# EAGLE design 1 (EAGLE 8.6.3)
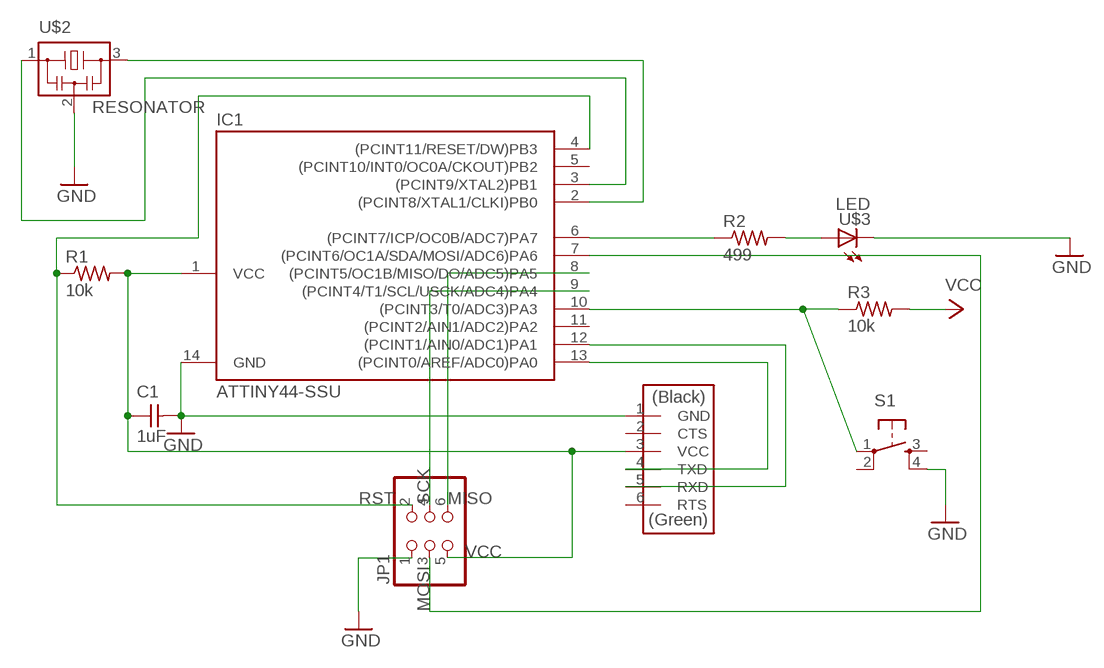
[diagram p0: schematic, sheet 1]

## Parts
C1  1uF  CAP-UNPOLARIZEDFAB  [C1206FAB]
IC1  ATTINY44-SSU  [SOIC14]
JP1  PINHD-2X3-SMD  [2X03SMD]
R1  10k  RES-US1206FAB  [R1206FAB]
R2  499  RES-US1206FAB  [R1206FAB]
R3  10k  RES-US1206FAB  [R1206FAB]
S1  6MM_SWITCH6MM_SWITCH  [6MM_SWITCH]
U$1  FTDI-SMD-HEADER  [1X06SMD]
U$2  RESONATOR  [EFOBM]
U$3  LED  [LED1206]

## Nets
GND: C1.2 IC1.14(GND) JP1.1 S1.4(S1) U$1.1(GND) U$2.2 U$3.2(C)
MISO: IC1.8((PCINT5/OC1B/MISO/DO/ADC5)PA5) JP1.6
MOSI: IC1.7((PCINT6/OC1A/SDA/MOSI/ADC6)PA6) JP1.3
N$1: IC1.2((PCINT8/XTAL1/CLKI)PB0) U$2.3
N$2: IC1.3((PCINT9/XTAL2)PB1) U$2.1
N$4: IC1.13((PCINT0/AREF/ADC0)PA0) U$1.4(TXD)
N$5: IC1.12((PCINT1/AIN0/ADC1)PA1) U$1.5(RXD)
N$6: IC1.6((PCINT7/ICP/OC0B/ADC7)PA7) R2.1
N$7: R2.2 U$3.1(A)
N$8: IC1.10((PCINT3/T0/ADC3)PA3) R3.1 S1.1(P)
RST: IC1.4((PCINT11/RESET/DW)PB3) JP1.2 R1.1
SCK: IC1.9((PCINT4/T1/SCL/USCK/ADC4)PA4) JP1.4
VCC: C1.1 IC1.1(VCC) JP1.5 R1.2 R3.2 U$1.3(VCC)
Unconnected: IC1.5((PCINT10/INT0/OC0A/CKOUT)PB2) IC1.11((PCINT2/AIN1/ADC2)PA2) S1.2(P1) S1.3(S) U$1.2(CTS) U$1.6(RTS)

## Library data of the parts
C1 = fab:CAP-UNPOLARIZED
IC1 = fab:ATTINY44
JP1 = fab:PINHD-2X3-SMD: PIN HEADER
R1-R3 = fab:RES-US: Resistor (US Symbol)
S1 = fab:6MM_SWITCH: OMRON SWITCH
U$1 = fab:FTDI-SMD-HEADER
U$2 = fab:RESONATOR
U$3 = fab:LED: LED

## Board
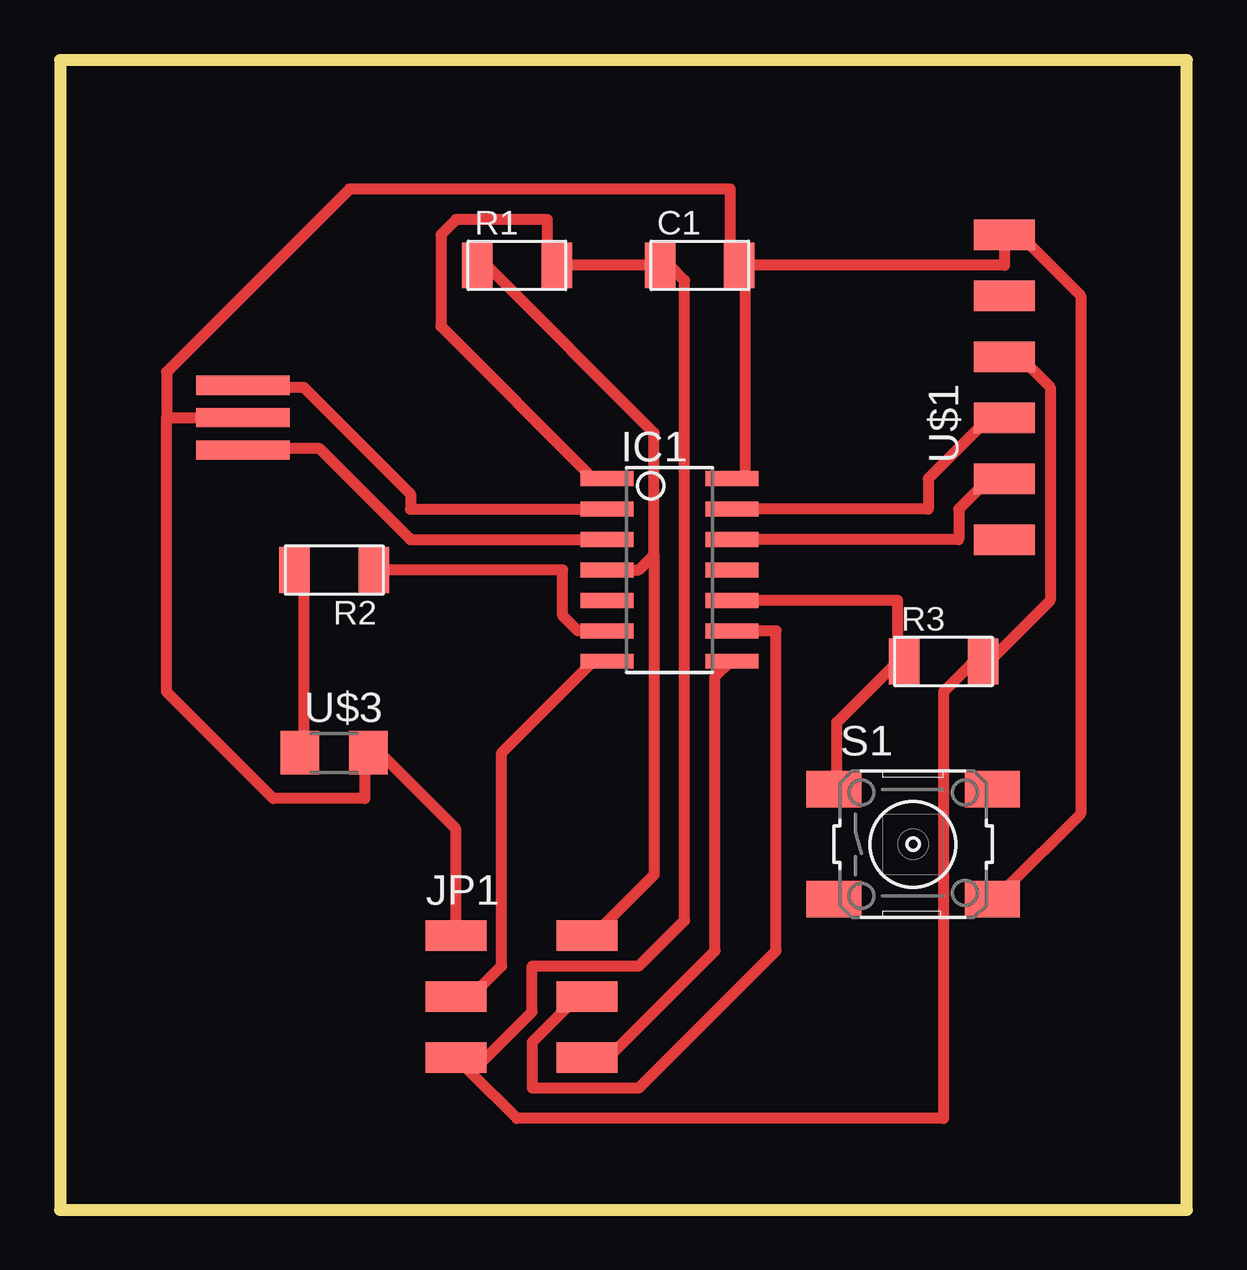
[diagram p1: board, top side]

Size 46.97 x 47.93 mm. Coordinates in mm from the lower left corner, seen from the top.
Outline: 0,0 46.97,0 46.97,47.93 0,47.93 0,0
Copper layers (1*16): Top 0.035mm / dielectric 1.5mm / Bottom 0.035mm
Design rules "default *": minimum track width 16mil, minimum drill 0.35mm, track to track 16mil, track to pad 16mil, pad to pad 16mil, via to via 16mil, smd to smd 16mil, copper to edge 40mil, drill to drill 6mil, minimum pad ring 10mil, minimum via ring 8mil, stop-mask expansion 4mil, vias tented up to drill 0mil, thermal gap 10mil

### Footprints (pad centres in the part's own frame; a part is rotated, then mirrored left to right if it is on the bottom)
C1206FAB = smd 1.27 x 1.905: 1 -1.651,0; 2 1.651,0
SOIC14 = smd 0.61 x 2.21: 1 -3.81,-2.603; 2 -2.54,-2.603; 3 -1.27,-2.603; 4 0,-2.603; 5 1.27,-2.603; 6 2.54,-2.603; 7 3.81,-2.603; 8 3.81,2.603; 9 2.54,2.603; 10 1.27,2.603; 11 0,2.603; 12 -1.27,2.603; 13 -2.54,2.603; 14 -3.81,2.603
2X03SMD = smd 2.54 x 1.27: 1 -2.54,2.54; 2 2.92,2.54; 3 -2.54,0; 4 2.92,0; 5 -2.54,-2.54; 6 2.92,-2.54
R1206FAB = smd 1.27 x 1.905: 1 -1.651,0; 2 1.651,0
6MM_SWITCH = smd 2.286 x 1.524: 1 -3.302,2.286; 2 3.302,2.286; 3 -3.302,-2.286; 4 3.302,-2.286
1X06SMD = smd 2.54 x 1.27: 1 0,6.35; 2 0,3.81; 3 0,1.27; 4 0,-1.27; 5 0,-3.81; 6 0,-6.35
EFOBM = smd 0.8 x 3.9: 1 -1.35,0; 2 0,0; 3 1.35,0
LED1206 = smd 1.6 x 1.803: 1 -1.422,0; 2 1.422,0

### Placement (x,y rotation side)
C1  26.67,39.37 0 top
IC1  25.4,26.67 270 top
JP1  19.05,8.89 0 top
R1  19.05,39.37 0 top
R2  11.43,26.67 180 top
R3  36.83,22.86 0 top
S1  35.56,15.24 0 top
U$1  39.37,34.29 0 top
U$2  7.62,33.02 90 top
U$3  11.43,19.05 0 top

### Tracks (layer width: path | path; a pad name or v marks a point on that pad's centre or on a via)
GND
  Top 0.457: JP1.1 16.51,15.88 13.33,19.05 U$3.2 12.7,19.05 12.7,17.15 8.89,17.15 4.45,21.59 4.45,33.02 | 4.45,33.02 U$2.2 | 28.57,39.37 28.57,30.48 IC1.14 | S1.4 39.37,13.33 42.55,16.51 42.55,38.1 40,40.64 U$1.1 39.37,39.37 28.57,39.37 | 28.57,39.37 C1.2 27.94,39.37 27.94,42.55 12.06,42.55 4.45,34.92 4.45,33.02
MISO
  Top 0.457: JP1.6 22.86,6.35 27.3,10.79 27.3,22.23 27.94,22.86 IC1.8
MOSI
  Top 0.457: JP1.3 17.14,8.89 18.41,10.16 18.41,19.05 22.23,22.86 IC1.7
N$1
  Top 0.457: IC1.2 14.6,29.21 14.6,29.84 10.16,34.29 7.62,34.29 U$2.3
N$2
  Top 0.457: IC1.3 14.6,27.94 10.79,31.75 7.62,31.75 U$2.1
N$4
  Top 0.457: IC1.13 36.2,29.21 36.2,30.48 38.73,33.02 U$1.4
N$5
  Top 0.457: IC1.12 37.46,27.94 37.46,29.21 38.73,30.48 U$1.5
N$6
  Top 0.457: R2.1 20.95,26.67 20.95,24.77 21.59,24.13 IC1.6
N$7
  Top 0.457: U$3.1 10.16,19.05 10.16,26.67 R2.2
N$8
  Top 0.457: 34.92,22.86 32.38,20.32 32.38,17.78 S1.1 | IC1.10 34.92,25.4 34.92,22.86 | 34.92,22.86 R3.1
RST
  Top 0.457: 24.77,27.3 24.77,32.38 17.78,39.37 R1.1 | 24.77,27.3 24.13,26.67 IC1.4 | 24.77,27.3 24.77,13.97 22.23,11.43 JP1.2
SCK
  Top 0.457: IC1.9 29.84,24.13 29.84,10.79 24.13,5.08 19.69,5.08 19.69,6.99 21.59,8.89 JP1.4
VCC
  Top 0.457: IC1.1 22.23,30.48 15.88,36.83 15.88,40.64 16.51,41.27 20.32,41.27 20.32,39.37 R1.2 C1.1 25.4,39.37 26.03,38.73 26.03,12.06 24.13,10.16 19.69,10.16 19.69,8.26 17.14,5.71 | U$1.3 40,35.56 41.27,34.29 41.27,25.4 38.73,22.86 R3.2 38.1,22.86 36.83,21.59 36.83,3.81 19.05,3.81 17.14,5.71 | 17.14,5.71 JP1.5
